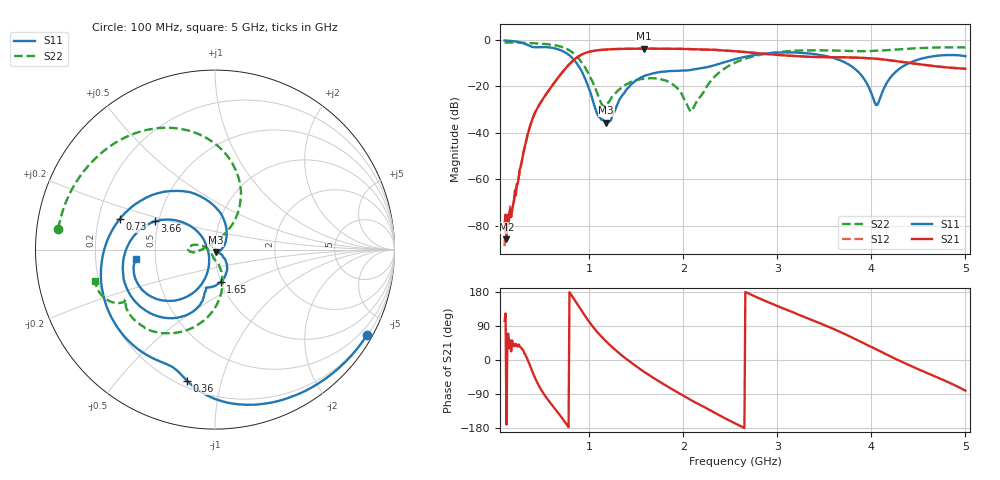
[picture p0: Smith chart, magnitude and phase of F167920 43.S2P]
!  2-Port S-parameters saved by WinCal
! VAR MeasName=S-Parameters (CALIBRATED_DATA) read from VNA (N5242A)
! VAR MeasDate=2016-11-22 9:57:37
! VAR NAME=F167920 43
! VAR FILENAME=F167920 43.S2P
! VAR DATE=2016-11-22 9:57:37
! VAR PHYS_PORTS=1,2
# Hz S DB R 50
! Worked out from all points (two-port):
!   491 points, 100 MHz to 5 GHz, reference 50 ohm
!   highest |S21| = -3.73 dB at 1.58 GHz (marker M1); lowest = -85.9 dB at 120 MHz (marker M2)
!   |S21| within 3 dB of the highest: 902.1 MHz to 3.086 GHz (2.184 GHz wide, 110 % of centre)
!   lowest |S11| = -35.7 dB at 1.18 GHz (marker M3), VSWR 1.03, Z = 50.3 - j1.61 ohm
!   |S11| at or under -10 dB: 865.3 MHz to 2.407 GHz (1.542 GHz wide, 94.2 % of centre); 3.732 GHz to 4.401 GHz (668.1 MHz wide, 16.4 % of centre)
!   |S22| runs from -30.9 to -1.1 dB; largest |S21 - S12| = 0.0012
!   S11 on the Smith chart (normalised r, x): 100 MHz: 0.22, -3.82; 360 MHz: 0.24, -0.78; 730 MHz: 0.29, +0.14; 1.65 GHz: 0.99, -0.37; 3.66 GHz: 0.48, +0.17; 5 GHz: 0.39, -0.05
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1e8  -0.25 -29.3  -79.15 103.4  -88.86 66.8  -1.10 172.4
1.2e8  -0.30 -35.0  -85.86 -170.4  -80.43 44.5  -1.11 170.8
1.9e8  -0.56 -55.1  -71.25 36.6  -72.13 43.5  -1.16 165.5
3.6e8  -2.52 -101.9  -38.58 -8.3  -38.44 -8.1  -1.36 151.3
6e8  -3.39 -155.3  -20.02 -117.5  -20.02 -117.5  -2.08 124.6
7.3e8  -5.09 162.0  -13.15 -159.6  -13.15 -159.7  -3.34 102.7
9.2e8  -13.51 82.6  -6.31 129.2  -6.31 129.2  -9.76 63.7
1.09e9  -32.35 -27.8  -4.48 72.6  -4.47 72.7  -23.61 67.8
1.18e9  -35.73 -77.4  -4.16 48.9  -4.15 48.9  -28.25 140.7
1.58e9  -15.62 -72.2  -3.73 -30.6  -3.73 -30.5  -16.77 -177.9
1.65e9  -14.72 -80.3  -3.77 -42.1  -3.77 -42.0  -16.46 179.6
1.74e9  -13.92 -89.6  -3.79 -56.1  -3.79 -56.1  -16.72 174.3
1.93e9  -13.35 -101.2  -3.86 -84.1  -3.85 -84.0  -20.53 164.2
2.08e9  -12.96 -102.9  -3.97 -105.5  -3.96 -105.5  -30.88 -146.5
2.55e9  -8.32 -111.6  -4.88 -167.2  -4.88 -167.2  -9.82 -89.9
3.37e9  -5.99 -178.1  -7.31 105.4  -7.31 105.3  -4.49 -139.8
3.66e9  -8.66 154.8  -7.49 75.1  -7.49 75.1  -4.66 -148.4
3.89e9  -15.06 135.5  -7.70 47.9  -7.71 47.9  -4.87 -150.7
4.05e9  -28.05 -174.8  -8.11 28.3  -8.11 28.4  -4.70 -150.1
4.19e9  -16.89 -108.4  -8.74 10.9  -8.74 10.9  -4.37 -150.6
4.5e9  -8.47 -130.7  -10.47 -24.5  -10.47 -24.5  -3.56 -155.2
5e9  -7.03 -173.3  -12.44 -80.9  -12.44 -81.0  -3.24 -165.4
